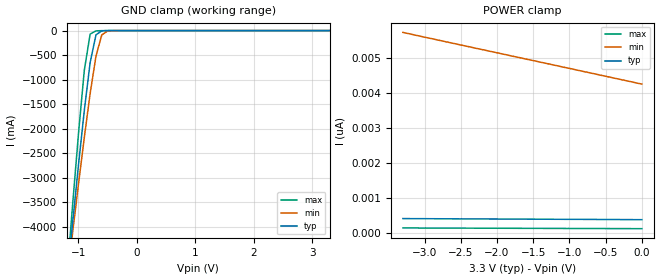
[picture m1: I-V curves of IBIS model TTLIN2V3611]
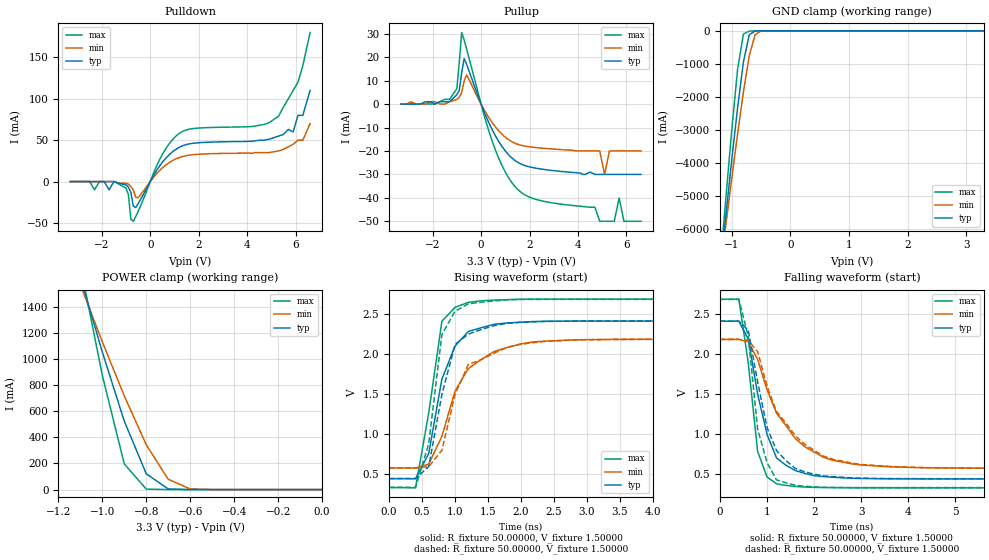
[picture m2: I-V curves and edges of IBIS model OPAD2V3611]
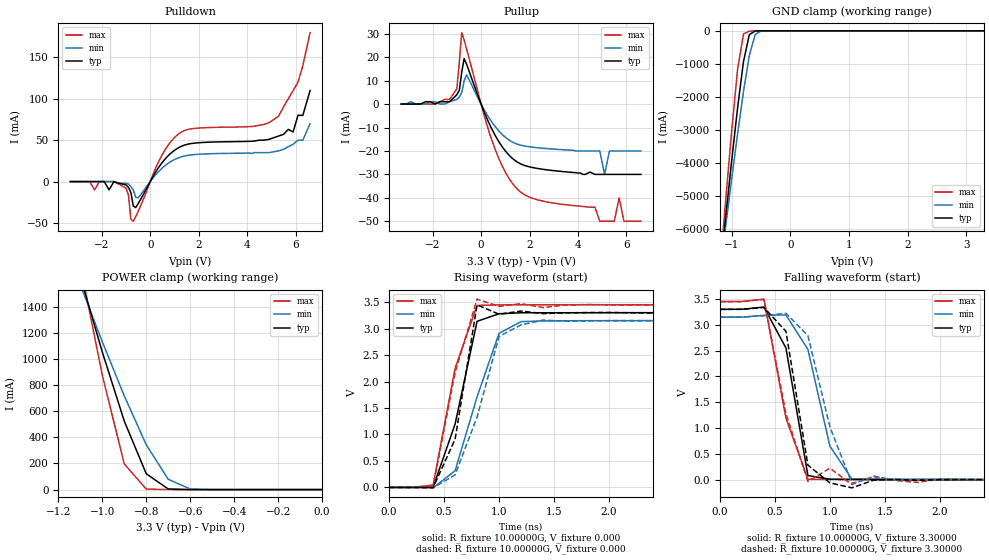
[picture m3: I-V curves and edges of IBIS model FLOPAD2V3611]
| IBIS file 36110pf.ibs created by s2ibis2 version 1.2
| North Carolina State University Electronics Research Laboratory  1995
[IBIS ver]   2.1
[File name]   72v36110p.ibs
[File Rev]   1.0
[Date]   Friday, April 4, 2003
[Source]   IDT
[Notes]   1. Temp typ=25C, min=-40C, max=85C
   2. IDT C11_5_3.3V_SAC_2M process
   3. Ramp rates based on 50 ohm load
[Disclaimer]
READ THESE TERMS AND CONDITIONS CAREFULLY BEFORE USING THIS IBIS MODEL.  BY
USING THIS IBIS MODEL, YOU ARE ACCEPTING AND AGREEING TO THESE TERMS AND
CONDITIONS OF USE.
Integrated Device Technology, Inc. ("IDT") hereby grants the user of this
IBIS model ("User") a non-exclusive, nontransferable license to use this
IBIS model under the following terms: The User is granted this license only
to use the IBIS model for demonstration purposes only and is not granted
rights to sell, copy (except as needed to run the IBIS model), rent, lease
or sub-license (except for demonstration) the IBIS model in whole or in
part, or in modified form to anyone. The User may modify the IBIS model to
suit its specific applications, but  rights to derivative works and such
modifications shall belong to IDT.
THIS IBIS MODEL IS PROVIDED ON AN AS IS" BASIS AND IDT  MAKES ABSOLUTELY NO
WARRANTY WITH RESPECT TO THE INFORMATION CONTAINED HEREIN.  IDT DISCLAIMS
AND USER WAIVES ALL WARRANTIES, EXPRESS AND IMPLIED, INCLUDING WARRANTIES OF
MERCHANTABILITY AND FITNESS FOR A PARTICULAR PURPOSE.  THE ENTIRE RISK AS TO
QUALITY AND PERFORMANCE IS WITH THE USER  ACCORDINGLY, IN NO EVENT SHALL IDT
BE LIABLE FOR ANY DIRECT OR INDIRECT DAMAGES, WHETHER IN CONTRACT OR TORT,
INCLUDING ANY LOST PROFITS OR OTHER INCIDENTAL, CONSEQUENTIAL, EXEMPLARY, OR
PUNITIVE DAMAGES ARISING OUT OF THE USE OR APPLICATION OF THE  IBIS MODEL,
WHETHER OR NOT IDT HAD NOTICE OF SUCH DAMAGES.
IDT reserves the right to make changes without notice to any product herein
to improve reliability, function, or design. IDT does not convey any license
under patent rights or any other intellectual property rights, including
those of third parties. IDT is not obligated to provide maintenance or
support for the licensed IBIS model.
This model is for the 3.3v High-Density Supersync II 36-Bit FIFO
[Copyright]
Copyright 2002, Integrated Device Technology, Inc. All rights reserved.
|   Component 72V36110PF
[Component]   72V36110PF
[Manufacturer]   Integrated Device Technology Inc.
[Package]
|Following package parameters are for 128 lead TQFP package
| variable   typ   min   max
R_pkg   0.18500   0.15800   0.25500
L_pkg   8.85000nH   5.51000nH   13.23000nH
C_pkg   0.24200pF   0.12100pF   0.36700pF
[Pin]  signal_name   model_name   R_pin   L_pin   C_pin
1   /WEN   TTLIN2V3611
2   /SEN   TTLIN2V3611
3   NC   NC
4   VCC   POWER
5   NC   NC
6   IW   TTLIN2V3611
7   D35   TTLIN2V3611
8   D34   TTLIN2V3611
9   D33   TTLIN2V3611
10   D32   TTLIN2V3611
11   VCC   POWER
12   D31   TTLIN2V3611
13   D30   TTLIN2V3611
14   GND   GND
15   D29   TTLIN2V3611
16   D28   TTLIN2V3611
17   D27   TTLIN2V3611
18   D26   TTLIN2V3611
19   D25   TTLIN2V3611
20   D24   TTLIN2V3611
21   D23   TTLIN2V3611
22   GND   GND
23   D22   TTLIN2V3611
24   VCC   POWER
25   D21   TTLIN2V3611
26   D20   TTLIN2V3611
27   D19   TTLIN2V3611
28   D18   TTLIN2V3611
29   GND   GND
30   D17   TTLIN2V3611
31   D16   TTLIN2V3611
32   D15   TTLIN2V3611
33   D14   TTLIN2V3611
34   D13   TTLIN2V3611
35   VCC   POWER
36   D12   TTLIN2V3611
37   GND   GND
38   D11   TTLIN2V3611
39   D10   TTLIN2V3611
40   D9   TTLIN2V3611
41   D8   TTLIN2V3611
42   D7   TTLIN2V3611
43   D6   TTLIN2V3611
44   GND   GND
45   D5   TTLIN2V3611
46   D4   TTLIN2V3611
47   D3   TTLIN2V3611
48   VCC   POWER
49   D2   TTLIN2V3611
50   D1   TTLIN2V3611
51   D0   TTLIN2V3611
52   GND   GND
53   Q0   OPAD2V3611
54   Q1   OPAD2V3611
55   Q2   OPAD2V3611
56   Q3   OPAD2V3611
57   Q4   OPAD2V3611
58   Q5   OPAD2V3611
59   GND   GND
60   Q6   OPAD2V3611
61   VCC   POWER
62   Q7   OPAD2V3611
63   Q8   OPAD2V3611
64   Q9   OPAD2V3611
65   Q10   OPAD2V3611
66   Q11   OPAD2V3611
67   GND   GND
68   Q12   OPAD2V3611
69   Q13   OPAD2V3611
70   Q14   OPAD2V3611
71   Q15   OPAD2V3611
72   VCC   POWER
73   VCC   POWER
74   Q16   OPAD2V3611
75   Q17   OPAD2V3611
76   GND   GND
77   Q18   OPAD2V3611
78   Q19   OPAD2V3611
79   Q20   OPAD2V3611
80   Q21   OPAD2V3611
81   Q22   OPAD2V3611
82   Q23   OPAD2V3611
83   GND   GND
84   GND   GND
85   Q24   OPAD2V3611
86   Q25   OPAD2V3611
87   VCC   POWER
88   Q26   OPAD2V3611
89   Q27   OPAD2V3611
90   Q28   OPAD2V3611
91   Q29   OPAD2V3611
92   Q30   OPAD2V3611
93   Q31   OPAD2V3611
94   GND   GND
95   GND   GND
96   Q32   OPAD2V3611
97   Q33   OPAD2V3611
98   Q34   OPAD2V3611
99   Q35   OPAD2V3611
100   VCC   POWER
101   VCC   POWER
102   /OE   TTLIN2V3611
103   /RT   TTLIN2V3611
104   /REN   TTLIN2V3611
105   RCLK   TTLIN2V3611
106   GND   GND
107   RM   TTLIN2V3611
108   /EF/OR   FLOPAD2V3611
109   PFM   TTLIN2V3611
110   /PAE   FLOPAD2V3611
111   VCC   POWER
112   BM   TTLIN2V3611
113   IP   TTLIN2V3611
114   /BE   TTLIN2V3611
115   FS1   TTLIN2V3611
116   GND   GND
117   /HF   FLOPAD2V3611
118   FS0   TTLIN2V3611
119   OW   TTLIN2V3611
120   GND   GND
121   /PAF   FLOPAD2V3611
122   VCC   POWER
123   /FF-/IR   FLOPAD2V3611
124   FWFT/SI   TTLIN2V3611
125   /LD   TTLIN2V3611
126   /MRS   TTLIN2V3611
127   /PRS   TTLIN2V3611
128   WCLK   TTLIN2V3611
| Models and submodels in the file (3): TTLIN2V3611 (Input), OPAD2V3611 (3-state), FLOPAD2V3611 (3-state)
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| in   in   dummy_model
| oe   oe   dummy_model
| in1  in1   dummy_model
| oe1  oe1   dummy_model
|   Model TTLIN2V3611
[Model]   TTLIN2V3611
Model_type   Input
Polarity   Non-Inverting
Vinl =  0.80000V
Vinh =  2.00000V
C_comp   10.00000pF   10.00000pF   10.00000pF
[Temperature Range]   25.00000   85.00000   -40.00000
[Voltage Range]   3.30000V   3.15000V   3.45000V
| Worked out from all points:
|   GND clamp passes 1 mA (typ) near -0.51 V on its own axis
[GND_clamp]
| voltage   I(typ)   I(min)   I(max)
-3.3V     -31.62A    -27.14A    -38.3A
-1.2V     -5.12A     -5.123A    -5.052A
-1.1V     -3.918A    -4.12A     -3.553A
-1V       -2.746A    -3.136A    -2.109A
-900mV    -1.631A    -2.183A    -811.7mA
-800mV    -652.4mA   -1.286A    -71.19mA
-700mV    -87.47mA   -520.5mA   -5.646mA
-600mV    -5.364mA   -87.77mA   -1.458mA
-500mV    -302uA     -8.09mA    -219uA
3.3V      373pA      4.31nA     115.1pA
[POWER_clamp]
| voltage   I(typ)   I(min)   I(max)
-3.3V     403.8pA    5.719nA    136.4pA
-2.6V     396.7pA    5.404nA    131.5pA
-1.3V     385pA      4.825nA    123.6pA
0V        373pA      4.243nA    116pA
|   Model OPAD2V3611
[Model]   OPAD2V3611
Model_type   3-state
Polarity   Non-Inverting
Enable   Active-High
Vmeas =  1.50000V
C_comp   10.00000pF   10.00000pF   10.00000pF
[Temperature Range]   25.00000   85.00000   -40.00000
[Voltage Range]   3.30000V   3.15000V   3.45000V
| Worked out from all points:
|   slope of the pulldown table from 0 to 0.495 V, typ, clamps not added: 21.5 ohm
|   slope of the pullup table from 0 to 0.495 V, typ, clamps not added: 42.4 ohm
|   GND clamp passes 1 mA (typ) near -0.52 V on its own axis
|   POWER clamp passes 1 mA (typ) near -0.62 V on its own axis
|   rising waveform, R_fixture 50.00000, V_fixture 1.50000: 20-80 % time 343ps typ, 520ps min, 265ps max; typ from 0.444 V to 2.42 V
|   rising waveform, R_fixture 50.00000, V_fixture 1.50000: 20-80 % time 313ps typ, 368ps min, 223ps max; typ from 0.447 V to 2.42 V
|   falling waveform, R_fixture 50.00000, V_fixture 1.50000: 20-80 % time 461ps typ, 858ps min, 278ps max; typ from 2.42 V to 0.444 V
|   falling waveform, R_fixture 50.00000, V_fixture 1.50000: 20-80 % time 485ps typ, 875ps min, 322ps max; typ from 2.42 V to 0.447 V
[Pulldown]
| voltage   I(typ)   I(min)   I(max)
-3.3V     0A         0A         0A
-1V       -4mA       -2mA       -8mA
-800mV    -13.1mA    -6mA       -45.44mA
-700mV    -29.4mA    -10mA      -47.99mA
-500mV    -26.74mA   -19.63mA   -36.09mA
400mV     19.36mA    13.74mA    27.32mA
1.2V      41.38mA    29.07mA    58.2mA
5.3V      55mA       37mA       79mA
5.9V      60mA       45mA       110mA
6.1V      80mA       50mA       120mA
6.3V      80mA       50mA       140mA
6.6V      110mA      70mA       180mA
[Pullup]
| voltage   I(typ)   I(min)   I(max)
-3.3V     0A         0A         0A
-1.3V     1mA        1mA        2mA
-1V       4mA        2mA        6.6mA
-800mV    13.4mA     4.9mA      30.49mA
-600mV    17.05mA    12.41mA    23.59mA
500mV     -11.77mA   -8.469mA   -17mA
1.5V      -24.75mA   -17.12mA   -36.28mA
4.9V      -30mA      -20mA      -50mA
5.1V      -30mA      -30mA      -50mA
5.7V      -30mA      -20mA      -40mA
5.9V      -30mA      -20mA      -50mA
6.6V      -30mA      -20mA      -50mA
[GND_clamp]
| voltage   I(typ)   I(min)   I(max)
-3.3V     -44.86A    -38.5A     -54.32A
-1.2V     -7.292A    -7.294A    -7.196A
-1.1V     -5.587A    -5.872A    -5.069A
-1V       -3.924A    -4.477A    -3.02A
-900mV    -2.338A    -3.123A    -1.172A
-800mV    -940.2mA   -1.846A    -98.36mA
-700mV    -115.7mA   -749mA     -8.05mA
-600mV    -4.278mA   -114.8mA   -2.238mA
-500mV    -295.2uA   -5.816mA   -325.4uA
3.3V      607.7pA    5.602nA    92.71pA
[POWER_clamp]
| voltage   I(typ)   I(min)   I(max)
-3.3V     15.46A     11.9A      22.55A
-1.1V     1.627A     1.567A     1.714A
-1V       1.053A     1.131A     875.2mA
-900mV    523.9mA    716.9mA    196.8mA
-800mV    121.2mA    343.1mA    4.087mA
-700mV    5.031mA    78.95mA    112.4uA
-600mV    111.5uA    5.081mA    8.814uA
0V        607.7pA    2.814nA    110.2pA
[Ramp]
| variable   typ   min   max
dV/dt_r   0.80040/0.49852n   0.55518/0.74186n   1.11420/0.33285n
dV/dt_f   1.24980/0.73875n   0.95160/1.28926n   1.51836/0.39958n
R_load = 50.00000
[Rising Waveform]
R_fixture = 50.00000
V_fixture = 1.50000
V_fixture_min = 1.50000
V_fixture_max = 1.50000
| time   V(typ)   V(min)   V(max)
0s        444.1mV    577.5mV    332.7mV
400ps     443.2mV    577.5mV    329.4mV
600ps     759mV      626.9mV    1.268V
800ps     1.69V      974.8mV    2.415V
1ns       2.105V     1.542V     2.588V
1.2ns     2.286V     1.821V     2.651V
1.6ns     2.377V     2.039V     2.679V
2ns       2.402V     2.131V     2.689V
2.4ns     2.414V     2.167V     2.69V
10ns      2.417V     2.189V     2.691V
[Rising Waveform]
R_fixture = 50.00000
V_fixture = 1.50000
V_fixture_min = 1.50000
V_fixture_max = 1.50000
R_dut = 0.18500
L_dut = 8.85000nH
C_dut = 0.24200pF
| time   V(typ)   V(min)   V(max)
0s        446.7mV    579.4mV    336mV
400ps     446.6mV    579.4mV    335.6mV
600ps     594.9mV    594.1mV    881.8mV
800ps     1.498V     800.6mV    2.25V
1ns       2.124V     1.499V     2.54V
1.2ns     2.253V     1.873V     2.632V
1.8ns     2.389V     2.09V      2.683V
2.2ns     2.407V     2.147V     2.688V
2.8ns     2.416V     2.179V     2.688V
10ns      2.416V     2.188V     2.688V
[Falling Waveform]
R_fixture = 50.00000
V_fixture = 1.50000
V_fixture_min = 1.50000
V_fixture_max = 1.50000
| time   V(typ)   V(min)   V(max)
0s        2.417V     2.189V     2.691V
400ps     2.417V     2.189V     2.692V
600ps     2.192V     2.159V     1.896V
800ps     1.502V     1.937V     786.7mV
1ns       1V         1.557V     467.2mV
1.2ns     707.2mV    1.267V     383.9mV
1.8ns     513.6mV    846.8mV    342.6mV
2.2ns     473.3mV    714.4mV    336.7mV
2.8ns     452.6mV    633mV      333.3mV
10ns      444.1mV    577.6mV    332.7mV
[Falling Waveform]
R_fixture = 50.00000
V_fixture = 1.50000
V_fixture_min = 1.50000
V_fixture_max = 1.50000
R_dut = 0.18500
L_dut = 8.85000nH
C_dut = 0.24200pF
| time   V(typ)   V(min)   V(max)
0s        2.416V     2.188V     2.688V
400ps     2.416V     2.188V     2.688V
600ps     2.305V     2.177V     2.226V
800ps     1.654V     2.034V     1.067V
1ns       1.086V     1.605V     645.6mV
1.2ns     799.8mV    1.288V     433.5mV
1.6ns     575.7mV    982.2mV    364.9mV
2ns       502.9mV    801.7mV    346mV
3ns       454.2mV    625mV      336.4mV
10ns      446.7mV    579.4mV    336mV
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|   Model FLOPAD2V3611
[Model]   FLOPAD2V3611
Model_type   3-state
Polarity   Non-Inverting
Enable   Active-High
Vmeas =  1.50000V
C_comp   10.00000pF   10.00000pF   10.00000pF
[Temperature Range]   25.00000   85.00000   -40.00000
[Voltage Range]   3.30000V   3.15000V   3.45000V
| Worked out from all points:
|   slope of the pulldown table from 0 to 0.495 V, typ, clamps not added: 21.5 ohm
|   slope of the pullup table from 0 to 0.495 V, typ, clamps not added: 42.4 ohm
|   GND clamp passes 1 mA (typ) near -0.52 V on its own axis
|   POWER clamp passes 1 mA (typ) near -0.62 V on its own axis
|   rising waveform, R_fixture 10.00000G, V_fixture 0.000: 20-80 % time 239ps typ, 290ps min, 227ps max; typ from 0 V to 3.3 V
|   rising waveform, R_fixture 10.00000G, V_fixture 0.000: 20-80 % time 191ps typ, 284ps min, 222ps max; typ from 0 V to 3.29 V
|   falling waveform, R_fixture 10.00000G, V_fixture 3.30000: 20-80 % time 175ps typ, 205ps min, 221ps max; typ from 3.3 V to 0 V
|   falling waveform, R_fixture 10.00000G, V_fixture 3.30000: 20-80 % time 153ps typ, 241ps min, 225ps max; typ from 3.3 V to 0 V
[Pulldown]
| voltage   I(typ)   I(min)   I(max)
-3.3V     0A         0A         0A
-1V       -4mA       -2mA       -8mA
-800mV    -13.1mA    -6mA       -45.44mA
-700mV    -29.4mA    -10mA      -47.99mA
-500mV    -26.74mA   -19.63mA   -36.09mA
400mV     19.36mA    13.74mA    27.32mA
1.2V      41.38mA    29.07mA    58.2mA
5.3V      55mA       37mA       79mA
5.9V      60mA       45mA       110mA
6.1V      80mA       50mA       120mA
6.3V      80mA       50mA       140mA
6.6V      110mA      70mA       180mA
[Pullup]
| voltage   I(typ)   I(min)   I(max)
-3.3V     0A         0A         0A
-1.3V     1mA        1mA        2mA
-1V       4mA        2mA        6.6mA
-800mV    13.4mA     4.9mA      30.49mA
-600mV    17.05mA    12.41mA    23.59mA
500mV     -11.77mA   -8.469mA   -17mA
1.5V      -24.75mA   -17.12mA   -36.28mA
4.9V      -30mA      -20mA      -50mA
5.1V      -30mA      -30mA      -50mA
5.7V      -30mA      -20mA      -40mA
5.9V      -30mA      -20mA      -50mA
6.6V      -30mA      -20mA      -50mA
[GND_clamp]
| voltage   I(typ)   I(min)   I(max)
-3.3V     -44.86A    -38.5A     -54.32A
-1.2V     -7.292A    -7.294A    -7.196A
-1.1V     -5.587A    -5.872A    -5.069A
-1V       -3.924A    -4.477A    -3.02A
-900mV    -2.338A    -3.123A    -1.172A
-800mV    -940.2mA   -1.846A    -98.36mA
-700mV    -115.7mA   -749mA     -8.05mA
-600mV    -4.278mA   -114.8mA   -2.238mA
-500mV    -295.2uA   -5.816mA   -325.4uA
3.3V      607.7pA    5.602nA    92.71pA
[POWER_clamp]
| voltage   I(typ)   I(min)   I(max)
-3.3V     15.46A     11.9A      22.55A
-1.1V     1.627A     1.567A     1.714A
-1V       1.053A     1.131A     875.2mA
-900mV    523.9mA    716.9mA    196.8mA
-800mV    121.2mA    343.1mA    4.086mA
-700mV    5.031mA    78.95mA    112.4uA
-600mV    111.5uA    5.081mA    8.814uA
0V        607.7pA    2.814nA    110.2pA
[Ramp]
| variable   typ   min   max
dV/dt_r   0.80040/0.24935n   0.55518/0.34835n   1.11420/0.17021n
dV/dt_f   1.24980/0.48363n   0.95160/0.80240n   1.51836/0.26104n
R_load = 50.00000
[Rising Waveform]
R_fixture = 10.00000G
V_fixture = 0.000
V_fixture_min = 0.000
V_fixture_max = 0.000
| time   V(typ)   V(min)   V(max)
0s        0V         0V         0V
200ps     -592.5uV   -37.45uV   -1.019mV
400ps     3.601mV    -8.441mV   43.48mV
600ps     1.197V     314.4mV    2.251V
800ps     3.137V     1.711V     3.438V
1ns       3.28V      2.91V      3.448V
1.2ns     3.298V     3.131V     3.449V
1.8ns     3.299V     3.149V     3.45V
10ns      3.3V       3.15V      3.45V
[Rising Waveform]
R_fixture = 10.00000G
V_fixture = 0.000
V_fixture_min = 0.000
V_fixture_max = 0.000
R_dut = 0.18500
L_dut = 8.85000nH
C_dut = 0.24200pF
| time   V(typ)   V(min)   V(max)
0s        0V         0V         0V
400ps     -4.386mV   -7.905mV   16.31mV
600ps     910.4mV    235.9mV    2.172V
800ps     3.447V     1.331V     3.556V
1ns       3.271V     2.851V     3.419V
1.2ns     3.331V     3.069V     3.47V
1.4ns     3.283V     3.16V      3.397V
1.6ns     3.296V     3.139V     3.444V
1.8ns     3.303V     3.143V     3.454V
10ns      3.295V     3.15V      3.445V
[Falling Waveform]
R_fixture = 10.00000G
V_fixture = 3.30000
V_fixture_min = 3.15000
V_fixture_max = 3.45000
| time   V(typ)   V(min)   V(max)
0s        3.3V       3.15V      3.45V
200ps     3.301V     3.15V      3.453V
400ps     3.345V     3.183V     3.498V
600ps     2.552V     3.192V     1.191V
800ps     79.6mV     2.525V     8.023mV
1ns       8.737mV    647.8mV    3.594mV
1.2ns     4.579mV    12.73mV    1.742mV
10ns      2.865uV    0V         3.049uV
[Falling Waveform]
R_fixture = 10.00000G
V_fixture = 3.30000
V_fixture_min = 3.15000
V_fixture_max = 3.45000
R_dut = 0.18500
L_dut = 8.85000nH
C_dut = 0.24200pF
| time   V(typ)   V(min)   V(max)
0s        3.3V       3.15V      3.45V
400ps     3.336V     3.176V     3.492V
600ps     2.873V     3.224V     1.279V
800ps     281.7mV    2.79V      -33.24mV
1ns       -62.17mV   1.024V     222.2mV
1.2ns     -159mV     -71.51mV   -94.98mV
1.4ns     -8.63mV    43.76mV    68.6mV
1.8ns     -13mV      639uV      -53.81mV
2ns       450.6uV    8.769mV    13.19mV
10ns      227.6uV    -683.2uV   -9.519mV
